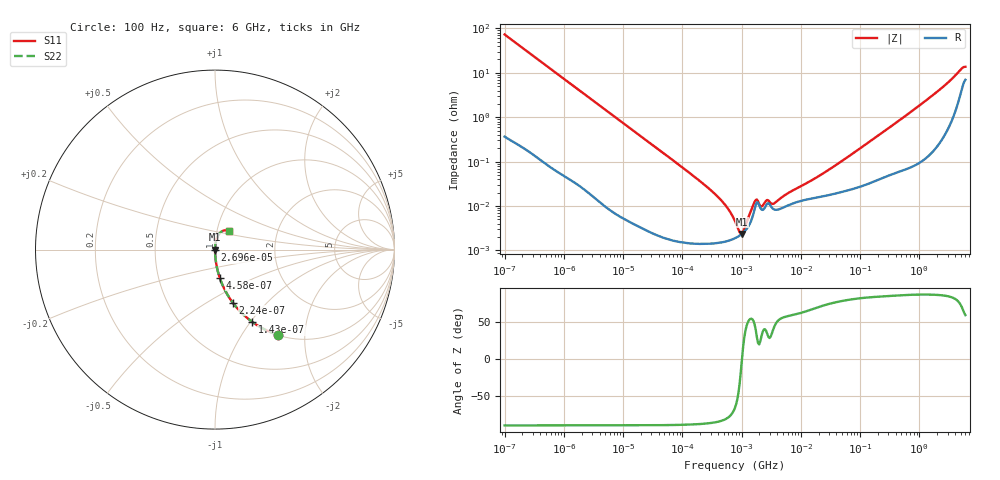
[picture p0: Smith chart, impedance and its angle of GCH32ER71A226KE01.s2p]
!Murata Part Number: GCH32ER71A226KE01
!These Parameters are Measured in Series Mode Connection
!Data Generated on Mar 13, 2026
!  o--ll--o
!Port1  Port2
!  o------o
!Operation Temp=25[degC], DC Bias Voltage=0[V]
!Freq. Start=100[Hz] Stop=6[GHz] 401[Steps]
# Hz S RI R 50
!Freq.(Hz) S11(Real) S11(Imag) S21(Real) S21(Imag) S12(Real) S12(Imag) S22(Real) S22(Imag)
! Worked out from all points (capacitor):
!   401 points, 100 Hz to 6 GHz, reference 50 ohm
!   read as one part in series: C = 21.7 uF near 109 Hz
!   lowest |Z| = 2.37 mohm at 1.013 MHz (marker M1)
!   series resonance near 1.015 MHz, so ESL is about 1.1 nH
!   S11 on the Smith chart (normalised r, x): 100 Hz: 1.01, -1.46; 143 Hz: 1.01, -1.02; 224 Hz: 1.00, -0.66; 458 Hz: 1.00, -0.32; 26.96 kHz: 1.00, -0.01; 6 GHz: 1.14, +0.24
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100  0.3492 -0.4742  0.6508 0.4742  0.6508 0.4742  0.3492 -0.4742
143  0.2088 -0.4038  0.7912 0.4038  0.7912 0.4038  0.2088 -0.4038
224  0.0983 -0.2948  0.9017 0.2948  0.9017 0.2948  0.0983 -0.2948
458  0.026 -0.1562  0.974 0.1562  0.974 0.1562  0.026 -0.1562
2008  0.00161 -0.0368  0.9984 0.0368  0.9984 0.0368  0.00161 -0.0368
26957  3.44e-05 -0.00277  1 0.00277  1 0.00277  3.44e-05 -0.00277
40335  2.46e-05 -0.00185  1 0.00185  1 0.00185  2.46e-05 -0.00185
231233  1.42e-05 -0.000309  1 0.000309  1 0.000309  1.42e-05 -0.000309
541393  1.59e-05 -0.000101  1 0.000101  1 0.000101  1.59e-05 -0.000101
774597  1.89e-05 -4.2e-05  1 4.2e-05  1 4.2e-05  1.89e-05 -4.2e-05
1013323  2.37e-05 -2e-07  1 2e-07  1 2e-07  2.37e-05 -2e-07
1449809  4.66e-05 6.54e-05  1 -6.54e-05  1 -6.54e-05  4.66e-05 6.54e-05
1813585  0.000122 6.92e-05  0.9999 -6.92e-05  0.9999 -6.92e-05  0.000122 6.92e-05
2169299  8.35e-05 5e-05  0.9999 -5e-05  0.9999 -5e-05  8.35e-05 5e-05
2713602  0.000114 7.68e-05  0.9999 -7.68e-05  0.9999 -7.68e-05  0.000114 7.68e-05
3549919  8.38e-05 7.91e-05  0.9999 -7.91e-05  0.9999 -7.91e-05  8.38e-05 7.91e-05
6075234  0.000103 0.000166  0.9999 -0.000166  0.9999 -0.000166  0.000103 0.000166
1.555665e7  0.000149 0.000356  0.9999 -0.000356  0.9999 -0.000356  0.000149 0.000356
3.124326e8  0.000527 0.00584  0.9995 -0.00584  0.9995 -0.00584  0.000527 0.00584
3.065283e9  0.00908 0.0597  0.9909 -0.0597  0.9909 -0.0597  0.00908 0.0597
5.016141e9  0.0456 0.1052  0.9544 -0.1052  0.9544 -0.1052  0.0456 0.1052
6e9  0.0765 0.1017  0.9235 -0.1017  0.9235 -0.1017  0.0765 0.1017
